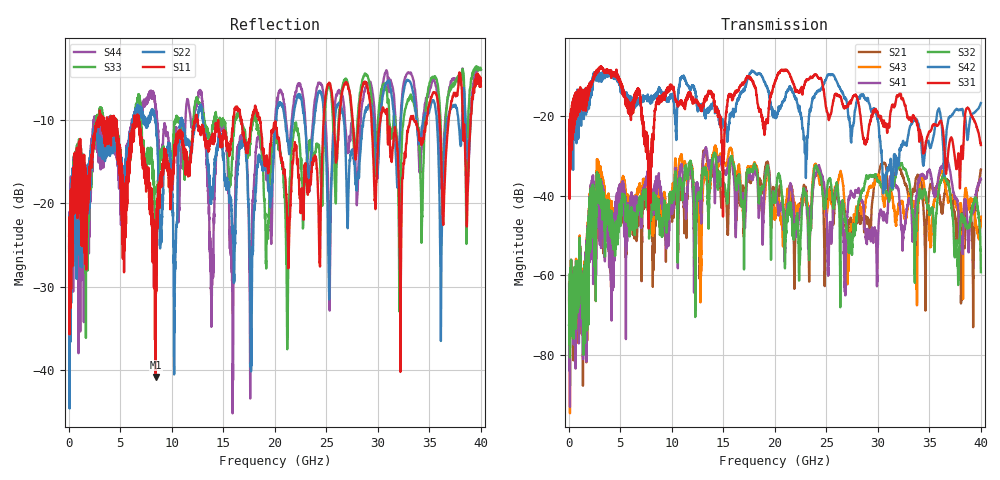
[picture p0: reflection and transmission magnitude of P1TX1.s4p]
!Agilent Technologies,N5245A,MY49151084,A.09.20.08
!Agilent N5245A: A.09.20.08
!Date: Thursday, March 01, 2012 11:46:28
!Correction: S11(Full 4 Port(1,2,3,4))
!S12(Full 4 Port(1,2,3,4))
!S13(Full 4 Port(1,2,3,4))
!S14(Full 4 Port(1,2,3,4))
!S21(Full 4 Port(1,2,3,4))
!S22(Full 4 Port(1,2,3,4))
!S23(Full 4 Port(1,2,3,4))
!S24(Full 4 Port(1,2,3,4))
!S31(Full 4 Port(1,2,3,4))
!S32(Full 4 Port(1,2,3,4))
!S33(Full 4 Port(1,2,3,4))
!S34(Full 4 Port(1,2,3,4))
!S41(Full 4 Port(1,2,3,4))
!S42(Full 4 Port(1,2,3,4))
!S43(Full 4 Port(1,2,3,4))
!S44(Full 4 Port(1,2,3,4))
!S4P File: Measurements: <S11,S12,S13,S14>,
!<S21,S22,S23,S24>,
!<S31,S32,S33,S34>,
!<S41,S42,S43,S44>:
# Hz S  dB  R 50
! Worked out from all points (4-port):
!   3996 points, 50 MHz to 40 GHz, reference 50 ohm
!   strongest paths, dB at 50 MHz, 10.04 GHz, 20.03 GHz, 30.02 GHz, 40 GHz:
!     S31: -23.6, -13.1, -11.4, -19.6, -27.2
!     S42: -27.1, -14.8, -20.0, -21.4, -16.7
!     S32: -72.6, -41.7, -41.8, -36.5, -59.3
!     S41: -62.2, -44.7, -38.8, -51.1, -35.8
!     S43: -66.0, -40.5, -45.1, -35.3, -45.3
!     S21: -64.1, -46.6, -38.0, -35.2, -33.5
!   lowest |S11| = -40.9 dB at 8.45 GHz (marker M1), VSWR 1.02, Z = 50.2 - j0.874 ohm
!   |S11| at or under -10 dB: start of sweep to 2.8 GHz; 6.824 GHz to 12.3 GHz (5.476 GHz wide, 57.3 % of centre); 18.57 GHz to 24.74 GHz (6.174 GHz wide, 28.5 % of centre)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
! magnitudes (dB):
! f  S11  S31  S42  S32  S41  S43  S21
! 50 MHz  -23.9  -23.6  -27.1  -72.6  -62.2  -66.0  -64.1
! 2.9 GHz  -10.3  -8.6  -10.4  -37.0  -36.5  -33.6  -40.1
! 8.45 GHz  -40.9  -18.1  -15.2  -41.7  -38.3  -41.0  -41.6
! 15.91 GHz  -11.1  -15.4  -19.8  -31.2  -32.3  -30.2  -31.5
! 26.79 GHz  -5.7  -17.8  -15.4  -45.8  -62.6  -43.3  -52.2
! 30.65 GHz  -8.8  -22.3  -36.4  -38.6  -45.0  -42.5  -31.8
! 40 GHz  -5.9  -27.2  -16.7  -59.3  -35.8  -45.3  -33.5
